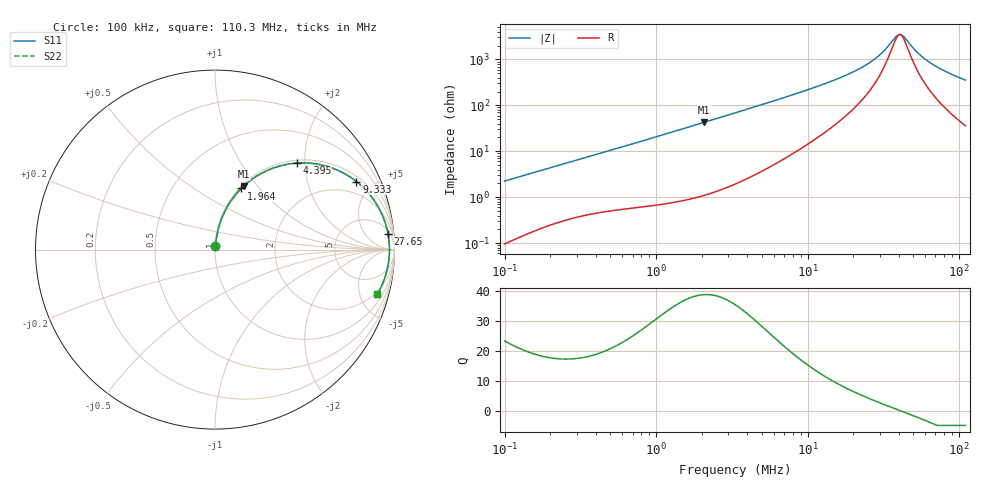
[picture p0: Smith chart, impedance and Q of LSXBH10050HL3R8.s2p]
! LSXBH10050HL3R8  S-PARAMETER MODEL  ( General Type )
! Model Generated by TAIYO YUDEN Corporation (http://www.ty-top.com)
! Version 3.0
! TAIYO YUDEN Control No. 180118NI43SB-FBB
! Copyright(c) 2007 TAIYO YUDEN CO.,LTD. All Rights Reserved.
! Product Description (link to TY-COMPAS)
! https://ds.yuden.co.jp/TYCOMPAS/or/detail?pn=LSXBH10050HL3R8N&u=M
! Products Name : Inductors
! Characteristics :
!  Inductance : 3.8 uH , SRF(min) : 26 MHz , DC Resistance(max) : 0.0169 Ohm
!  Rated Current : Saturation :7300 mA , Temp Rise : 6800 mA (40 degC)
!  Case Size : 10.0 x 9.8 / 0.394 x 0.386 [mm/inch] , Thickness : 5 / 0.197 [mm/inch]
!  (Conditions: Temperature = 25 degC , DC Bias Current/Voltage = 0A / 0V)
! External Node Assignments :
!  1  o---GGG---o  2
! GND o---------o GND
! Frequency Range : 0.1MHz  -  110.285862MHz  [ 402 STEP ]
# MHz S RI R 50
! Freq[MHz].  S11 Real  S11 Imag  S21 Real  S21 Imag  S12 Real  S12 Imag  S22 Real  S22 Imag
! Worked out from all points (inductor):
!   401 points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, 100 kHz to 110.3 MHz, reference 50 ohm
!   read as one part in series: L = 3.55 uH near 103.6 kHz
!   highest Q = 38.9 at 2.07 MHz (marker M1), where L = 3.27 uH
!   self-resonance near 40.72 MHz
!   S11 on the Smith chart (normalised r, x): 100 kHz: 1.00, +0.04; 1.964 MHz: 1.02, +0.81; 4.395 MHz: 1.06, +1.82; 9.333 MHz: 1.24, +4.02; 27.65 MHz: 7, +19; 110.3 MHz: 1.72, -7.05
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0.1  0.00147 0.0224  0.9985 -0.0224  0.9985 -0.0224  0.00147 0.0224
0.323312  0.00855 0.0681  0.9914 -0.0681  0.9914 -0.0681  0.00855 0.0681
0.607364  0.0209 0.123  0.9791 -0.123  0.9791 -0.123  0.0209 0.123
1.045308  0.0503 0.2031  0.9497 -0.2031  0.9497 -0.2031  0.0503 0.2031
1.963681  0.1464 0.3408  0.8536 -0.3408  0.8536 -0.3408  0.1464 0.3408
2.069616  0.1595 0.3535  0.8405 -0.3535  0.8405 -0.3535  0.1595 0.3535
3.320932  0.3238 0.454  0.6762 -0.454  0.6762 -0.454  0.3238 0.454
4.395019  0.4546 0.4819  0.5454 -0.4819  0.5454 -0.4819  0.4546 0.4819
6.238594  0.6257 0.4634  0.3743 -0.4634  0.3743 -0.4634  0.6257 0.4634
9.333222  0.7881 0.3793  0.2119 -0.3793  0.2119 -0.3793  0.7881 0.3793
10.73698  0.8307 0.3414  0.1693 -0.3414  0.1693 -0.3414  0.8307 0.3414
18.80544  0.935 0.1857  0.065 -0.1857  0.065 -0.1857  0.935 0.1857
23.2038  0.9538 0.1318  0.0462 -0.1318  0.0462 -0.1318  0.9538 0.1318
27.64535  0.9638 0.0892  0.0362 -0.0892  0.0362 -0.0892  0.9638 0.0892
31.25117  0.9683 0.0604  0.0317 -0.0604  0.0317 -0.0604  0.9683 0.0604
34.71395  0.9707 0.0363  0.0293 -0.0363  0.0293 -0.0363  0.9707 0.0363
39.24173  0.972 0.00835  0.028 -0.00835  0.028 -0.00835  0.972 0.00835
42.08946  0.9721 -0.00754  0.0279 0.00754  0.0279 0.00754  0.9721 -0.00754
52.85125  0.9685 -0.0596  0.0315 0.0596  0.0315 0.0596  0.9685 -0.0596
62.96776  0.9616 -0.1009  0.0384 0.1009  0.0384 0.1009  0.9616 -0.1009
81.88658  0.9428 -0.1665  0.0572 0.1665  0.0572 0.1665  0.9428 -0.1665
110.2859  0.9048 -0.2469  0.0952 0.2469  0.0952 0.2469  0.9048 -0.2469
